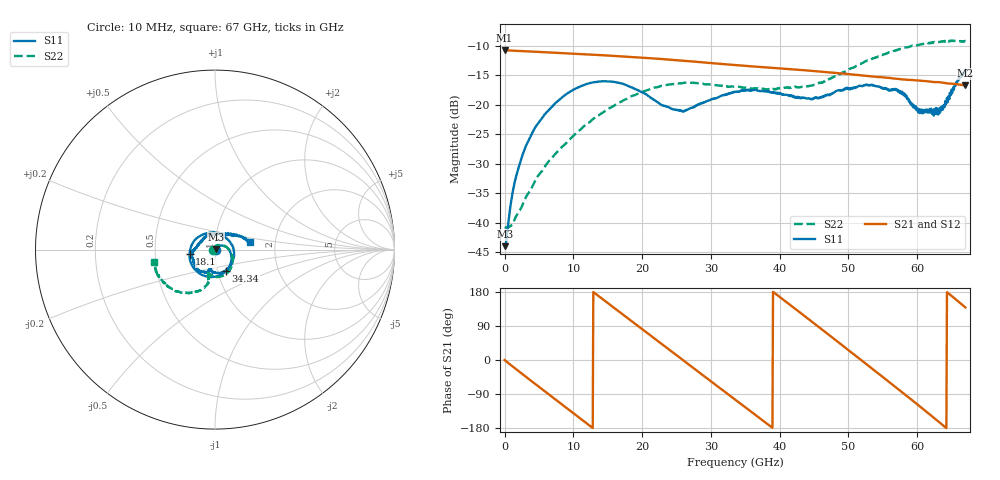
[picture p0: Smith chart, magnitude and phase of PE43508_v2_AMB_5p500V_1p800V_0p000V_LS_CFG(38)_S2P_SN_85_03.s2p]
!Keysight Technologies,N5227A,US51270237,A.10.43.00
!Date: Wednesday, August 22, 2018 17:10:31
!Correction: S11(Full 2 Port(1,3))
!S31(Full 2 Port(1,3))
!S13(Full 2 Port(1,3))
!S33(Full 2 Port(1,3))
!S2P File: Measurements: S11, S31, S13, S33:
# Hz S  dB  R 50
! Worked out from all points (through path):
!   801 points, 10 MHz to 67 GHz, reference 50 ohm
!   highest |S21| = -10.72 dB at 10 MHz (marker M1); lowest = -16.7 dB at 67 GHz (marker M2)
!   group delay of S21, straight-line fit = 38.7 ps
!   lowest |S11| = -44.0 dB at 93.74 MHz (marker M3), VSWR 1.01, Z = 50.6 + j0.0958 ohm
!   |S11| at or under -10 dB: start of sweep to end of sweep
!   |S22| runs from -40.9 to -9.1 dB; largest |S21 - S12| = 0.0016
!   S11 on the Smith chart (normalised r, x): 10 MHz: 1.01, -0.00; 18.1 GHz: 0.75, -0.04; 34.34 GHz: 1.10, -0.26; 67 GHz: 1.47, +0.13
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1e7  -43.73 -3.8  -10.72 -0.2  -10.72 -0.2  -40.85 -179.3
9.37375e7  -44.01 8.6  -10.73 -1.5  -10.74 -1.5  -40.85 175.8
1.601012e9  -32.51 47.0  -10.82 -23.1  -10.82 -23.1  -39.09 122.2
3.69445e9  -25.60 22.8  -10.94 -52.6  -10.94 -52.6  -34.62 82.3
7.295162e9  -19.82 -25.6  -11.14 -102.9  -11.14 -102.8  -28.45 47.3
1.123082e10  -16.76 -78.6  -11.37 -157.4  -11.38 -157.4  -23.99 15.3
1.441285e10  -15.99 -120.4  -11.58 158.6  -11.58 158.6  -21.20 -6.8
1.80973e10  -16.88 -170.4  -11.84 107.7  -11.83 107.7  -18.75 -30.6
2.236791e10  -19.66 121.7  -12.18 48.7  -12.17 48.7  -16.93 -56.6
2.722469e10  -20.50 25.9  -12.63 -18.2  -12.63 -18.2  -16.25 -81.8
3.049045e10  -18.90 -22.8  -12.96 -63.0  -12.96 -63.0  -16.65 -94.3
3.3505e10  -17.82 -55.4  -13.24 -104.3  -13.24 -104.2  -16.93 -100.9
3.434238e10  -17.60 -62.8  -13.31 -115.7  -13.32 -115.6  -16.96 -101.6
3.936662e10  -18.04 -93.8  -13.75 175.2  -13.75 175.3  -17.41 -105.1
4.472582e10  -18.99 -104.5  -14.22 100.5  -14.21 100.6  -16.70 -103.4
5.067119e10  -17.20 -116.3  -14.86 16.5  -14.85 16.6  -13.69 -103.8
5.586291e10  -17.59 -154.1  -15.41 -57.4  -15.40 -57.7  -11.09 -120.0
5.787261e10  -18.25 -175.0  -15.67 -86.3  -15.68 -86.5  -10.39 -127.8
6.046848e10  -20.76 144.3  -15.91 -123.7  -15.91 -124.0  -9.73 -138.1
6.272939e10  -20.54 93.3  -16.14 -156.9  -16.14 -157.2  -9.33 -148.8
6.381798e10  -20.09 67.1  -16.24 -173.6  -16.28 -174.0  -9.21 -154.2
6.7e10  -14.04 12.6  -16.67 138.6  -16.74 138.6  -9.18 -168.8
